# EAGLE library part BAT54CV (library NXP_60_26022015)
Two Schottky barrier double diodes Two planar Schottky barrier double diodes with common cathodes and an integrated guard ring for stress protection encapsulated in a SOT666 ultra small and flat lead Surface-Mounted Device (SMD) plastic package. AAL Eindhoven MK
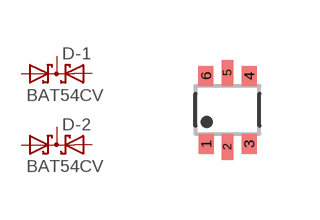
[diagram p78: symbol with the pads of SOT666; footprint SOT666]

Designator prefix D; gates -1=DIODE_SDD_AKKA -2=DIODE_SDD_AKKA

## BAT54CV  [SOT666]
1  -1:A1  pas
2  -1:A2  pas
3  -2:K1K2  pas
4  -2:A2  pas
5  -2:A1  pas
6  -1:K1K2  pas

## Footprint SOT666 (pad centres in mm)
SOT 666 Reflow soldering foorprint Source: Philips - BAS70_1PS7XSB70_SER_8.pdf
smd 0.375 x 0.5: 1 -0.537,-0.85; 3 0.538,-0.85; 4 0.538,0.85; 6 -0.538,0.85
smd 0.3 x 0.65: 2 0,-0.925; 5 0,0.925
